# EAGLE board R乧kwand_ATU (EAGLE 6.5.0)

No outline drawn. Coordinates in mm, seen from the top.
Copper layers (1*16): Top 0.035mm / dielectric 1.5mm / Bottom 0.035mm
Design rules "default": minimum track width 10mil, minimum drill 24mil, track to track 8mil, track to pad 8mil, pad to pad 8mil, via to via 8mil, smd to smd 8mil, copper to edge 40mil, drill to drill 8mil, minimum pad ring 10mil, minimum via ring 8mil, stop-mask expansion 4mil, vias tented up to drill 0mil, thermal gap 10mil

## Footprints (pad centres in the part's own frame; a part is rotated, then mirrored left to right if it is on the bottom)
SCHUBERT-FRONTPLATTE = hole 4: 7.084,10.746; 7.084,50.905; 183.949,10.746; 183.949,50.905
M25V = drill 1.016 octagon: 1 -16.561,1.422; 2 -13.792,1.422; 3 -11.049,1.422; 4 -8.28,1.422; 5 -5.512,1.422; 6 -2.769,1.422; 7 0,1.422; 8 2.769,1.422; 9 5.512,1.422; 10 8.28,1.422; 11 11.049,1.422; 12 13.792,1.422; 13 16.561,1.422; 14 -15.189,-1.422; 15 -12.421,-1.422; 16 -9.652,-1.422; 17 -6.909,-1.422; 18 -4.14,-1.422; 19 -1.372,-1.422; 20 1.372,-1.422; 21 4.14,-1.422; 22 6.909,-1.422; 23 9.652,-1.422; 24 12.421,-1.422; 25 15.189,-1.422 | hole 3.302: 23.52,0; -23.52,0
USB-VERLäNGERUNG = hole 3.2: -14,0; 14,0
SCHAFFNER_NETZANSCHLUSS = hole 3.2: -20,0; 20,0

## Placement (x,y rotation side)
E$1  [SCHUBERT-FRONTPLATTE]  0,0 0 top
E$2  [M25V]  134.54,52.07 180 top
E$3  [USB-VERLäNGERUNG]  73.12,52.07 0 top
E$4  [SCHAFFNER_NETZANSCHLUSS]  41.37,25.59 0 top

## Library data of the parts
E$1 E$3 E$4 = dk3ha-2020
E$2 = con-subd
